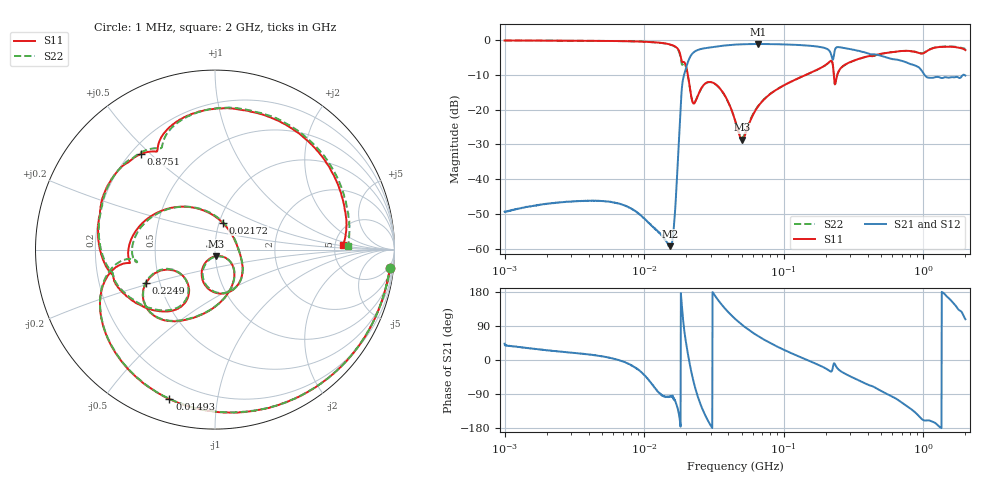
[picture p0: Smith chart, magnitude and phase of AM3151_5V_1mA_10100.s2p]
! Date/Time: Fri Jun 26 11:01:23 2020
! Network Analyzer:  Rev:
! Sweep from 1000000.0 to 2000000000.0, 1601 Points ! Power Supply: 0 V, 0 A
# HZ S DB R 50
!freq MagS11 AngS11 MagS21 AngS21 MagS12 AngS12 MagS22 AngS22
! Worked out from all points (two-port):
!   1601 points, 1 MHz to 2 GHz, reference 50 ohm
!   highest |S21| = -1.18 dB at 65.09 MHz (marker M1); lowest = -59.2 dB at 15.43 MHz (marker M2)
!   |S21| within 3 dB of the highest: 21.88 MHz to 218.3 MHz (196.5 MHz wide, 164 % of centre); 229.2 MHz to 453.4 MHz (224.2 MHz wide, 65.7 % of centre)
!   lowest |S11| = -28.6 dB at 50.36 MHz (marker M3), VSWR 1.08, Z = 50.5 - j3.69 ohm
!   |S11| at or under -10 dB: 20.55 MHz to 144.5 MHz (123.9 MHz wide, 150 % of centre); 228.3 MHz to 241.7 MHz (13.41 MHz wide, 5.71 % of centre)
!   |S22| runs from -28.1 to -0.2 dB; largest |S21 - S12| = 0.0076
!   S11 on the Smith chart (normalised r, x): 1 MHz: 3, -18; 14.93 MHz: 0.11, -0.73; 21.72 MHz: 1.04, +0.32; 224.9 MHz: 0.42, -0.19; 875.1 MHz: 0.24, +0.47; 2 GHz: 5.91, +0.64
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1000000  -0.16 -6.1  -49.24 43.0  -49.35 39.0  -0.17 -6.1
3555161  -0.26 -20.6  -46.14 16.7  -46.17 16.5  -0.26 -20.6
7748448  -0.39 -46.1  -48.03 -10.1  -47.96 -10.5  -0.40 -46.2
1.263916e7  -0.77 -83.1  -55.01 -85.2  -55.09 -84.5  -0.78 -83.4
1.492549e7  -1.20 -107.0  -59.08 -97.1  -58.81 -97.2  -1.24 -107.8
1.543016e7  -1.36 -113.4  -59.16 -95.9  -59.12 -96.1  -1.39 -114.5
1.649128e7  -1.80 -129.6  -51.66 -104.1  -51.38 -105.0  -1.88 -131.3
1.883746e7  -6.39 -171.3  -12.06 121.0  -12.04 120.9  -7.10 -170.8
2.003748e7  -7.91 152.4  -7.79 40.7  -7.78 40.7  -8.13 151.6
2.172285e7  -16.15 74.1  -4.35 -30.1  -4.35 -30.1  -16.23 70.1
2.446217e7  -15.55 -25.4  -2.82 -101.5  -2.83 -101.5  -15.56 -25.0
2.944137e7  -12.05 -75.9  -2.19 -168.1  -2.18 -168.1  -12.10 -74.2
4.493426e7  -23.29 -123.7  -1.35 108.1  -1.35 108.1  -23.25 -120.6
5.036085e7  -28.62 -79.7  -1.26 92.6  -1.26 92.5  -28.08 -77.6
6.508824e7  -19.21 -38.6  -1.18 63.6  -1.19 63.5  -19.12 -38.6
1.589914e8  -9.24 -96.2  -1.74 -5.3  -1.74 -5.3  -9.27 -96.3
2.248969e8  -7.36 -154.1  -5.69 -18.8  -5.66 -18.8  -7.28 -154.2
3.28878e8  -5.74 -143.2  -3.00 -50.5  -3.01 -50.2  -5.74 -144.2
5.652395e8  -3.64 171.7  -5.24 -92.1  -5.21 -92.0  -3.64 169.8
8.75068e8  -3.43 127.6  -7.38 -138.5  -7.35 -138.7  -3.41 125.2
1.393896e9  -1.99 73.9  -10.82 177.0  -10.81 176.8  -1.90 71.3
2e9  -2.93 2.1  -10.22 107.6  -10.38 107.1  -2.59 1.5
